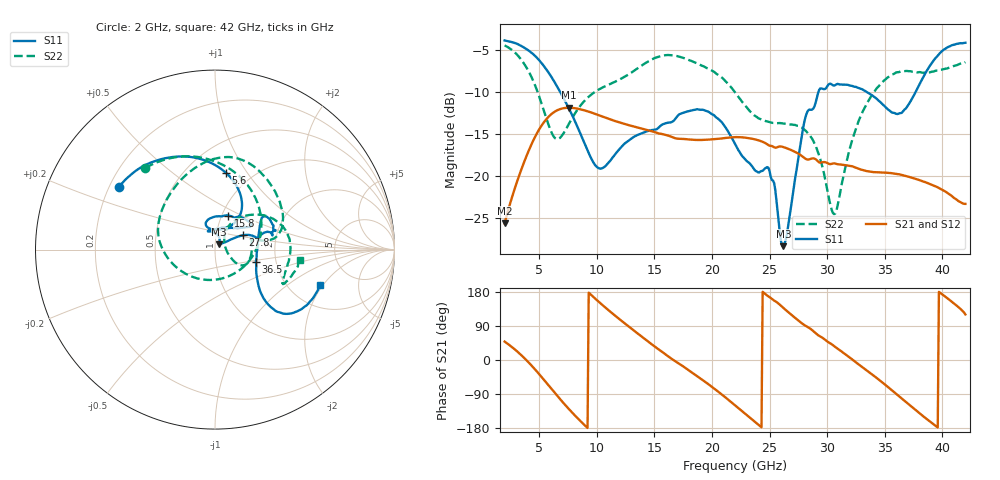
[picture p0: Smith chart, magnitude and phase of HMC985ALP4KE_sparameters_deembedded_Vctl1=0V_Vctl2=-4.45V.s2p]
!s2p File: Measurements: S11, S21, S12, S22
# GHz S dB R 50.0
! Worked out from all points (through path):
!   401 points, 2 GHz to 42 GHz, reference 50 ohm
!   highest |S21| = -11.89 dB at 7.6 GHz (marker M1); lowest = -25.7 dB at 2 GHz (marker M2)
!   lowest |S11| = -28.4 dB at 26.2 GHz (marker M3), VSWR 1.08, Z = 52.3 + j3.17 ohm
!   |S11| at or under -10 dB: 6.821 GHz to 29.25 GHz (22.43 GHz wide, 124 % of centre); 33.42 GHz to 37.69 GHz (4.272 GHz wide, 12 % of centre)
!   |S22| runs from -24.6 to -4.5 dB; largest |S21 - S12| = 0.0002
!   S11 on the Smith chart (normalised r, x): 2 GHz: 0.24, +0.28; 5.6 GHz: 0.76, +0.80; 15.8 GHz: 1.07, +0.42; 27.8 GHz: 1.34, +0.22; 36.5 GHz: 1.57, -0.23; 42 GHz: 2.94, -1.89
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2  -3.88 147.0  -25.66 48.6  -25.67 48.6  -4.47 130.5
3.6  -4.66 120.3  -18.70 8.4  -18.70 8.4  -6.47 84.9
4.7  -5.80 99.5  -15.21 -26.8  -15.22 -26.8  -9.42 43.4
5.6  -7.29 81.9  -13.29 -59.1  -13.30 -59.1  -13.05 -3.7
6.5  -9.22 66.5  -12.24 -92.0  -12.25 -92.0  -15.61 -69.0
7.6  -12.03 54.8  -11.89 -130.1  -11.90 -130.1  -13.77 -135.8
8.7  -15.38 55.1  -12.12 -164.7  -12.12 -164.7  -11.44 -170.2
10.4  -19.13 89.6  -12.90 147.5  -12.90 147.5  -9.56 162.4
15.4  -14.22 75.7  -14.97 27.5  -14.97 27.5  -5.80 87.1
15.8  -13.83 68.7  -15.07 18.6  -15.07 18.5  -5.67 82.0
19.4  -12.23 33.3  -15.71 -57.3  -15.72 -57.4  -7.05 35.0
22  -16.18 51.1  -15.40 -119.5  -15.40 -119.5  -10.06 9.9
24.9  -19.04 104.7  -16.34 167.8  -16.35 167.8  -13.57 13.2
26.2  -28.38 52.7  -16.58 137.4  -16.58 137.4  -13.78 -2.5
27.8  -15.23 27.2  -17.64 96.9  -17.64 96.9  -14.26 -24.5
28.7  -12.11 12.6  -17.94 78.8  -17.94 78.7  -15.60 -31.5
30.7  -9.21 20.8  -18.54 34.5  -18.54 34.5  -24.50 23.6
32.8  -9.58 33.9  -19.19 -13.1  -19.20 -13.1  -13.24 53.3
35.4  -12.21 11.7  -19.67 -74.3  -19.66 -74.3  -8.17 21.4
36.5  -12.47 -16.6  -19.91 -102.2  -19.91 -102.2  -7.54 7.3
39.5  -5.85 -43.7  -21.31 -175.7  -21.31 -175.7  -7.48 -26.3
42  -4.16 -18.6  -23.35 120.2  -23.34 120.2  -6.46 -7.2
